(* Logix 5000 AddOnInstructionDefinition export AMCI_3204_AOP_Run_Blend; software revision 20.03 *)

ADD_ON_INSTRUCTION AMCI_3204_AOP_Run_Blend   (* revision 1.0, vendor AMCI, ExecuteEnableInFalse *)
VAR_INPUT
   axis_status_bits : INT; {required}
   channel_number : INT; {required}
   Direction_0_for_CW_1_for_CCW : BOOL; {required}
END_VAR
VAR_IN_OUT
   AMCI_3204_output_data : AM:1756_3204:O:0; {required}
END_VAR
VAR_OUTPUT
   EN : BOOL; {access Read Only, visible}
   ER : BOOL; {access Read Only, visible}
END_VAR
VAR
   command_data_block : DINT[8]; {access None}
END_VAR

ROUTINE EnableInFalse   (* ladder *)
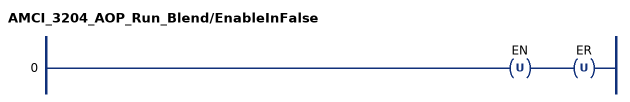
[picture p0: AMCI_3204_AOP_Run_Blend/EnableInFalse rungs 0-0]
   0: OTU(EN)OTU(ER);
END_ROUTINE

ROUTINE Logic   (* ladder *)
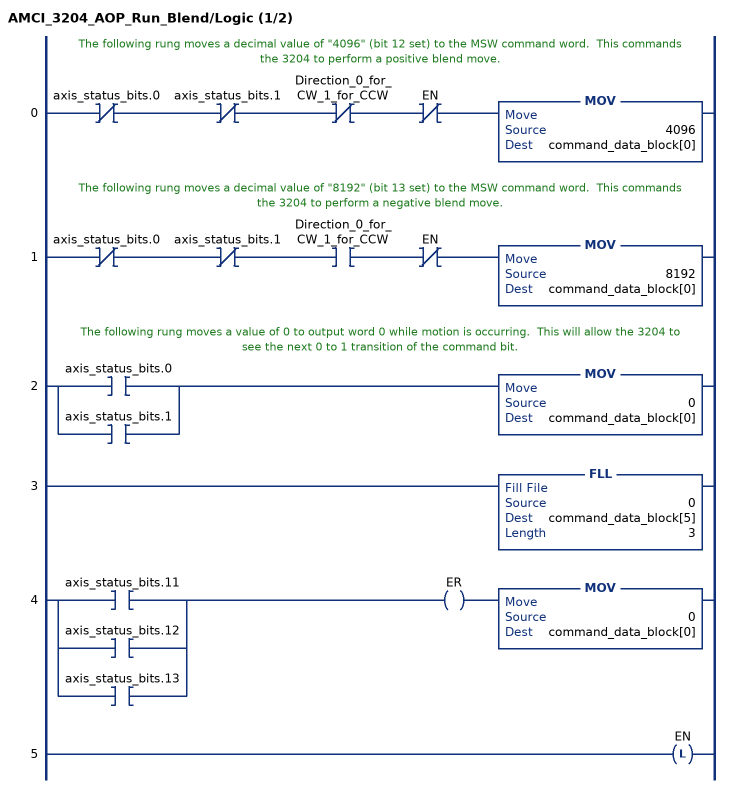
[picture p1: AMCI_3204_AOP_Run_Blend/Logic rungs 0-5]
   // The following rung moves a decimal value of "4096" (bit 12 set) to the MSW command word.  This commands the 3204 to perform a positive blend move.
   0: XIO(axis_status_bits.0)XIO(axis_status_bits.1)XIO(Direction_0_for_CW_1_for_CCW)XIO(EN)MOV(4096,command_data_block[0]);
   // The following rung moves a decimal value of "8192" (bit 13 set) to the MSW command word.  This commands the 3204 to perform a negative blend move.
   1: XIO(axis_status_bits.0)XIO(axis_status_bits.1)XIC(Direction_0_for_CW_1_for_CCW)XIO(EN)MOV(8192,command_data_block[0]);
   // The following rung moves a value of 0 to output word 0 while motion is occurring.  This will allow the 3204 to see the next 0 to 1 transition of the command bit.
   2: [XIC(axis_status_bits.0) ,XIC(axis_status_bits.1) ]MOV(0,command_data_block[0]);
   3: FLL(0,command_data_block[5],3);
   4: [XIC(axis_status_bits.11) ,XIC(axis_status_bits.12) ,XIC(axis_status_bits.13) ]OTE(ER)MOV(0,command_data_block[0]);
   5: OTL(EN);
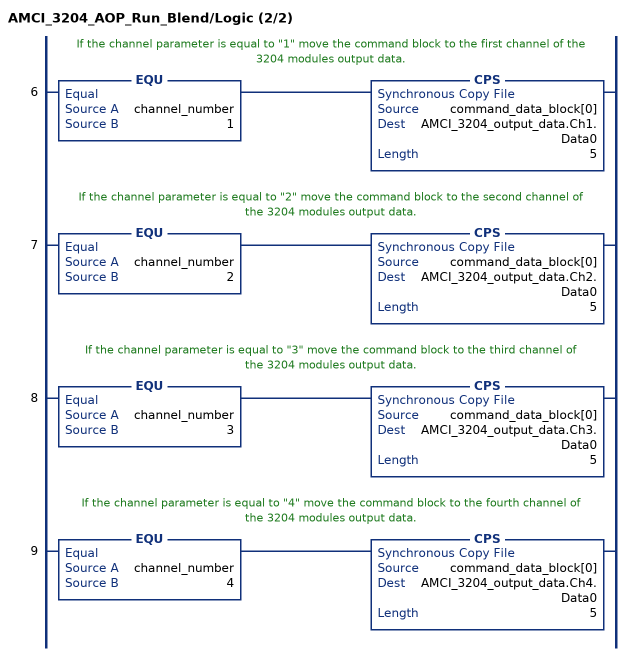
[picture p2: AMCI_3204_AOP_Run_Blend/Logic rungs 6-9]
   // If the channel parameter is equal to "1" move the command block to the first channel of the 3204 modules output data.
   6: EQU(channel_number,1)CPS(command_data_block[0],AMCI_3204_output_data.Ch1.Data0,5);
   // If the channel parameter is equal to "2" move the command block to the second channel of the 3204 modules output data.
   7: EQU(channel_number,2)CPS(command_data_block[0],AMCI_3204_output_data.Ch2.Data0,5);
   // If the channel parameter is equal to "3" move the command block to the third channel of the 3204 modules output data.
   8: EQU(channel_number,3)CPS(command_data_block[0],AMCI_3204_output_data.Ch3.Data0,5);
   // If the channel parameter is equal to "4" move the command block to the fourth channel of the 3204 modules output data.
   9: EQU(channel_number,4)CPS(command_data_block[0],AMCI_3204_output_data.Ch4.Data0,5);
END_ROUTINE
END_ADD_ON_INSTRUCTION
